{attribute 'call_after_init'}
FUNCTION_BLOCK FB_DS_IED_LD1_LLN0_DS1 EXTENDS FB_AcsiCommonDataSetClass
VAR
END_VAR

METHOD OnInit : BOOL
VAR
END_VAR
IF NOT DeleteAllMembers() THEN RETURN; END_IF
IF NOT AddMember(ipData:=fbIED.IEDLD1.LEDGGIO1.SPCSO1, eFc:=E_AcsiFc.ST_) THEN RETURN; END_IF
IF NOT AddMember(ipData:=fbIED.IEDLD1.LEDGGIO2.SPCSO1, eFc:=E_AcsiFc.ST_) THEN RETURN; END_IF
IF NOT AddMember(ipData:=fbIED.IEDLD1.LEDGGIO3.SPCSO1, eFc:=E_AcsiFc.ST_) THEN RETURN; END_IF
IF NOT AddMember(ipData:=fbIED.IEDLD1.LEDGGIO4.SPCSO1, eFc:=E_AcsiFc.ST_) THEN RETURN; END_IF
IF NOT AddMember(ipData:=fbIED.IEDLD1.LEDGGIO5.SPCSO1, eFc:=E_AcsiFc.ST_) THEN RETURN; END_IF
IF NOT AddMember(ipData:=fbIED.IEDLD1.LEDGGIO6.SPCSO1, eFc:=E_AcsiFc.ST_) THEN RETURN; END_IF
IF NOT AddMember(ipData:=fbIED.IEDLD1.LEDGGIO7.SPCSO1, eFc:=E_AcsiFc.ST_) THEN RETURN; END_IF
IF NOT AddMember(ipData:=fbIED.IEDLD1.LEDGGIO8.SPCSO1, eFc:=E_AcsiFc.ST_) THEN RETURN; END_IF
OnInit:= TRUE;
END_METHOD

END_FUNCTION_BLOCK
